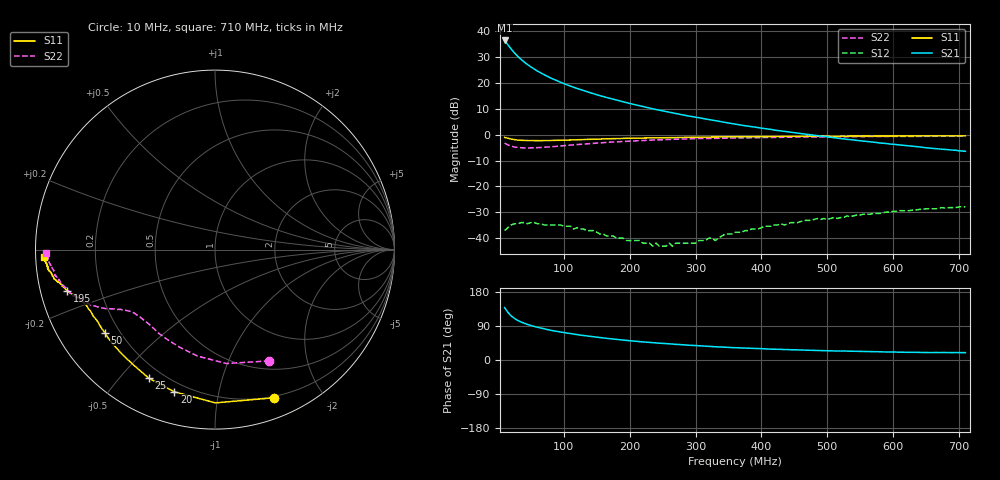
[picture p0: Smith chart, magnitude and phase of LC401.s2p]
!  POLYFET RF DEVICES
!  LC401
!  S PARAMETERS
!  VDS=28V, IDQ=250mA
! Date: Thu Jul 20 14:10:18 2000
! SCATTERING PARAMETERS :
# MHZ S MA R 50
!FREQ-MHZ MAG[S11] ANG[S11] MAG[S21] ANG[S21] MAG[S12] ANG[S12] MAG[S22] ANG[S22] MAG[S11] ANG[S11] MAG[S22] ANG[S22]
!  DEVICE  DEVICE  DEVICE  DEVICE  DEVICE  DEVICE  DEVICE  DEVICE  DEVICE  DEVICE  DEVICE  DEVICE
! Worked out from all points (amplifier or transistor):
!   141 points, 10 MHz to 710 MHz, reference 50 ohm
!   highest |S21| = 36.5 dB at 10 MHz (marker M1)
!   |S21| within 3 dB of that: start of sweep to 19 MHz
!   unconditionally stable (mu >= 1): 194.9073 MHz to 195.8304 MHz; 202.4 MHz to 382.6 MHz
!   at 125 MHz: K = 0.44, MSG = 27.0 dB, |S12| = -36.5 dB
!   at 360 MHz: K = 1.07, MAG = 19.2 dB, |S12| = -37.7 dB
!   at 710 MHz: K = 0.65, MSG = 10.8 dB, |S12| = -28.0 dB
!   S11 on the Smith chart (normalised r, x): 10 MHz: 0.19, -1.46; 20 MHz: 0.15, -0.74; 25 MHz: 0.15, -0.60; 50 MHz: 0.14, -0.33; 195 MHz: 0.08, -0.14; 710 MHz: 0.02, -0.02
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10  0.889 -68.2  66.58 138.2  0.014 44.7  0.69 -63.9
15  0.854 -89.8  54.91 125.7  0.016 38.2  0.638 -84.3
20  0.824 -106.0  45.38 116.2  0.018 28.2  0.601 -99.4
25  0.806 -117.2  38.24 109.7  0.019 24.4  0.578 -110.1
30  0.787 -125.2  32.82 104.4  0.019 19.6  0.567 -117.9
35  0.78 -131.4  28.59 100.2  0.02 14.1  0.562 -123.9
40  0.775 -136.1  25.38 96.8  0.02 12.2  0.556 -128.3
45  0.773 -140.1  22.64 93.7  0.019 11.5  0.555 -131.9
50  0.769 -143.1  20.46 91.0  0.02 7.6  0.557 -134.6
60  0.767 -147.9  16.99 86.3  0.019 3.4  0.563 -138.7
70  0.773 -151.2  14.51 82.3  0.018 0.9  0.572 -141.8
80  0.773 -153.6  12.52 78.3  0.018 -3.3  0.584 -143.9
95  0.781 -156.5  10.33 73.8  0.018 -4.6  0.607 -146.3
105  0.788 -157.9  9.2 71.1  0.017 -6.5  0.622 -147.6
130  0.809 -160.4  7.121 64.6  0.015 -5.5  0.663 -150.1
160  0.83 -162.5  5.46 58.2  0.012 -6.4  0.707 -152.5
195  0.854 -164.3  4.181 51.8  0.009 7.1  0.747 -155.2
245  0.876 -166.5  2.981 44.5  0.007 31.2  0.796 -159.1
360  0.914 -170.7  1.605 32.5  0.013 84.8  0.863 -166.2
480  0.938 -173.3  0.976 25.3  0.023 93.9  0.903 -171.8
595  0.946 -175.7  0.661 21.2  0.032 100.2  0.927 -175.6
710  0.952 -177.5  0.478 19.5  0.04 98.3  0.942 -178.9
